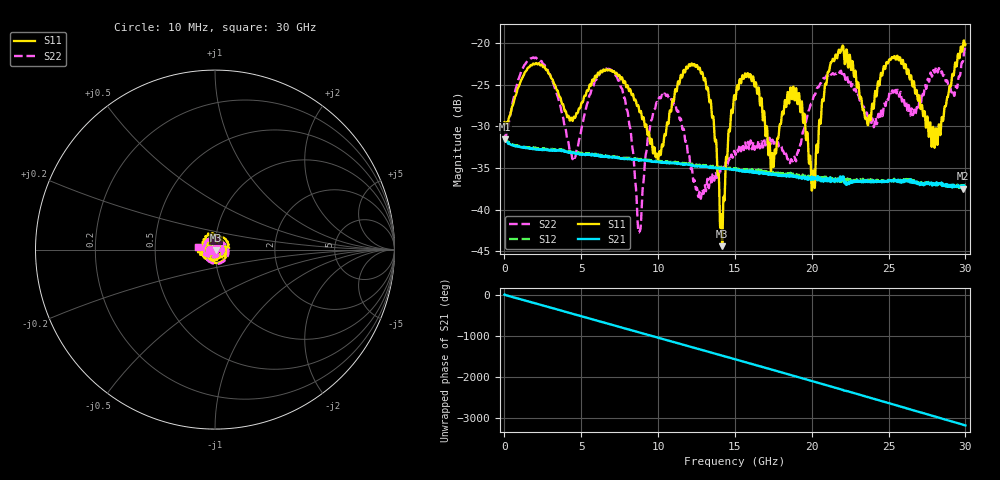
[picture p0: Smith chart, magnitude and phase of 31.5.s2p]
!Agilent Technologies,E8364B,US42250130,A.04.87.01
!Agilent E8364B: A.04.87.01
!Date: Monday, February 07, 2022 23:45:43
!Correction: S11(Full 2 Port SOLT,1,2) S21(Full 2 Port SOLT,1,2) S12(Full 2 Port SOLT,1,2) S22(Full 2 Port SOLT,1,2)
!S2P File: Measurements: S11, S21, S12, S22:
# Hz S  dB  R 50
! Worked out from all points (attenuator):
!   1601 points, 10 MHz to 30 GHz, reference 50 ohm
!   highest |S21| = -31.56 dB at 10 MHz (marker M1); lowest = -37.5 dB at 29.85 GHz (marker M2)
!   lowest |S11| = -44.4 dB at 14.18 GHz (marker M3), VSWR 1.01, Z = 50.4 - j0.427 ohm
!   |S11| at or under -10 dB: start of sweep to end of sweep
!   |S22| runs from -42.7 to -20.6 dB; largest |S21 - S12| = 0.0023
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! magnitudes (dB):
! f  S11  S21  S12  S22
! 10 MHz  -29.5  -31.6  -31.9  -31.6
! 1.903 GHz  -22.5  -32.7  -32.6  -21.7
! 4.377 GHz  -29.1  -33.1  -33.0  -33.4
! 5.015 GHz  -27.2  -33.4  -33.2  -30.2
! 7.208 GHz  -23.7  -33.7  -33.7  -23.8
! 8.107 GHz  -25.8  -33.9  -33.8  -29.5
! 8.782 GHz  -28.2  -34.1  -34.0  -42.7
! 10.02 GHz  -33.8  -34.2  -34.1  -26.8
! 12.61 GHz  -23.1  -34.8  -34.6  -38.4
! 13.51 GHz  -28.8  -34.9  -34.9  -36.5
! 14.18 GHz  -44.4  -35.1  -34.9  -35.1
! 15.01 GHz  -26.7  -35.2  -35.1  -33.2
! 16.26 GHz  -25.1  -35.6  -35.3  -32.6
! 17.44 GHz  -33.3  -35.7  -35.6  -31.6
! 18.9 GHz  -26.9  -36.0  -35.8  -33.9
! 20.01 GHz  -37.7  -36.0  -36.1  -27.1
! 21.43 GHz  -22.1  -36.3  -36.5  -23.7
! 23.7 GHz  -29.3  -36.7  -36.5  -29.0
! 25.01 GHz  -22.1  -36.5  -36.5  -26.5
! 28.09 GHz  -30.2  -37.1  -36.9  -22.9
! 29.85 GHz  -20.2  -37.5  -37.1  -22.1
! 30 GHz  -20.1  -37.3  -37.2  -20.6
